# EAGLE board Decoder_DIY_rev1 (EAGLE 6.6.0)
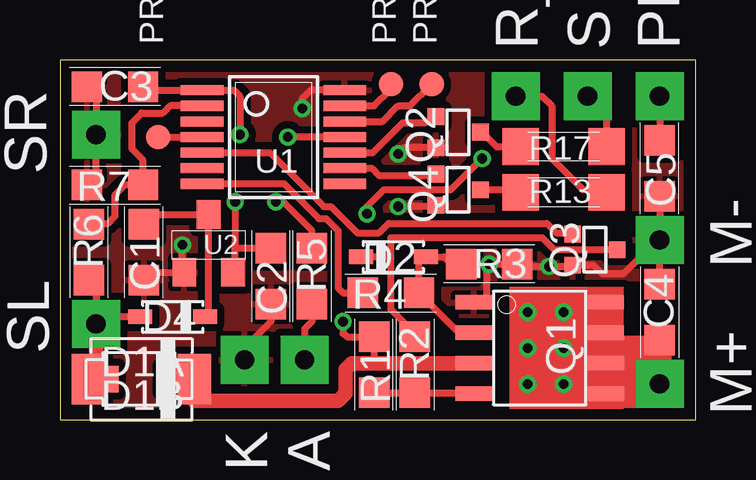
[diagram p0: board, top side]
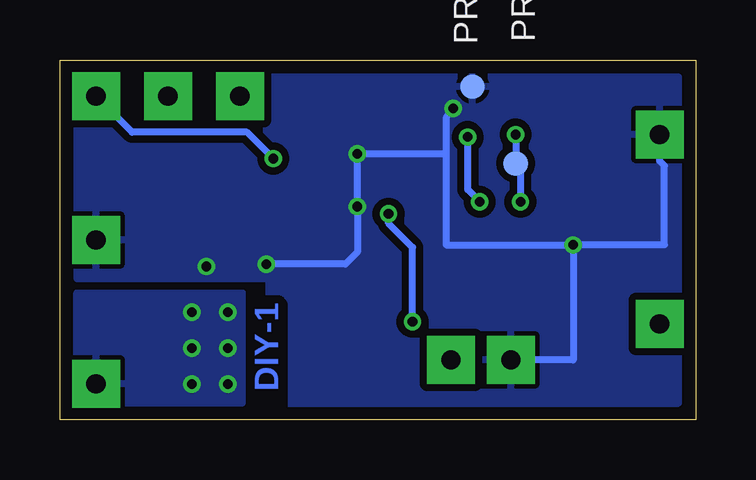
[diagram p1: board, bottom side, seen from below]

Size 26.5 x 15 mm. Coordinates in mm from the lower left corner, seen from the top.
Outline: 0,0 26.5,0 26.5,15 0,15 0,0
Copper layers (1*16): Top 0.035mm / dielectric 1.5mm / Bottom 0.035mm
Design rules "PCB-POOL Standard *": minimum track width 0.15mm, minimum drill 0.3mm, track to track 0.15mm, track to pad 0.15mm, pad to pad 0.15mm, via to via 0.15mm, smd to smd 0.15mm, copper to edge 0.3mm, drill to drill 0.2mm, minimum pad ring 0.2mm, minimum via ring 0.15mm, stop-mask expansion 0.075mm, vias tented up to drill 0.5mm, thermal gap 0.2mm
bRestrict: 2 lines

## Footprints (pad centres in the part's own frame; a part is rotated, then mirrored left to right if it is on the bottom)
LOETPAD_2X2_MM = drill 0.8 pad 2 square: P$1 0,0
0805 = smd 1.27 x 1.27: 1 -1.168,0; 2 1.168,0
SOD128 = smd 1.4 x 2.1: A -2.2,0; K 2.2,0
SOD123W = smd 1.1 x 1.1: A 1.4,0; K -1.4,0
SOD323 = smd 1 x 0.6: A 1.35,0; K -1.35,0
TESTPAD_RUND = smd 1.016 x 1.016: 1 0,0
SO8_COOLING = smd 0.61 x 1.524: 1 -1.905,-2.743; 2 -0.635,-2.743; 3 0.635,-2.743; 4 1.905,-2.743; 5 1.905,2.743; 6 0.635,2.743; 7 -0.635,2.743; 8 -1.905,2.743
SC70_FRANK = smd 0.7 x 0.7: 1 -0.65,-0.925; 2 0.65,-0.925; 3 0,0.925
1206 = smd 1.524 x 1.524: 1 1.792,0; 2 -1.79,0
TSSOP14 = smd 0.42 x 1.78: 1 -1.95,-2.97; 2 -1.3,-2.97; 3 -0.65,-2.97; 4 0,-2.97; 5 0.65,-2.97; 6 1.3,-2.97; 7 1.95,-2.97; 8 1.95,2.97; 9 1.3,2.97; 10 0.65,2.97; 11 0,2.97; 12 -0.65,2.97; 13 -1.3,2.97; 14 -1.95,2.97
SOT-23 = smd 0.991 x 1.194: 1 0,-1.27; 2 -1.016,1.143; 3 1.016,1.143

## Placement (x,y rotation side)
A  LOETPAD_2X2MM  [LOETPAD_2X2_MM]  10.2,2.5 0 top
C1  22u/16V/0805  [0805]  3.5,7 90 top
C2  100u/6,3V/0805  [0805]  8.8,6 90 top
C3  100n  [0805]  2.3,13.9 180 top
C4  100n  [0805]  25,4.5 270 top
C5  100n  [0805]  25,10.5 90 top
D1A  PMEG6030EP  [SOD128]  3.4,1.7 0 top
D1B  PMEG4020ER  [SOD123W]  3.3,1.7 180 top
D2  BAT760  [SOD323]  13.9,6.8 0 top
D4  BAT760  [SOD323]  4.7,4.3 180 top
K  LOETPAD_2X2MM  [LOETPAD_2X2_MM]  7.7,2.5 0 top
M+  LOETPAD_2X2MM  [LOETPAD_2X2_MM]  25,1.5 270 top
M-  LOETPAD_2X2MM  [LOETPAD_2X2_MM]  25,7.5 270 top
PLUS  LOETPAD_2X2MM  [LOETPAD_2X2_MM]  25,13.5 0 top
PROG_1  MCLR  [TESTPAD_RUND]  4.1,11.8 0 top
PROG_2  ICPDAT  [TESTPAD_RUND]  7.5,10.7 0 bottom
PROG_3  ICPDAT  [TESTPAD_RUND]  9.3,13.9 0 bottom
PROG_4  ICPDAT  [TESTPAD_RUND]  13.8,14 0 top
PROG_5  ICPCLK  [TESTPAD_RUND]  15.5,14 0 top
Q1  FDS8858CZ  [SO8_COOLING]  20,3 270 top
Q2  PDTC144EUA  [SC70_FRANK]  16.6,12 270 top
Q3  PDTC144EUA  [SC70_FRANK]  22.3,7.1 270 top
Q4  PDTC144EUA  [SC70_FRANK]  16.6,9.6 270 top
R1  1K  [0805]  13.1,2.3 90 top
R2  1K  [0805]  14.8,2.3 270 top
R3  18K  [0805]  17.9,6.5 180 top
R4  220R  [0805]  13.8,5.3 0 top
R5  390R  [0805]  10.5,6 270 top
R6  18K  [0805]  1.2,7 270 top
R7  10K  [0805]  2.3,9.8 0 top
R13  1K/1206  [1206]  21,9.5 180 top
R17  1K/1206  [1206]  21,11.4 180 top
R_B  LOETPAD_2X2MM  [LOETPAD_2X2_MM]  19,13.5 0 top
S  LOETPAD_2X2MM  [LOETPAD_2X2_MM]  22,13.5 0 top
SL  LOETPAD_2X2MM  [LOETPAD_2X2_MM]  1.5,4 0 top
SR  LOETPAD_2X2MM  [LOETPAD_2X2_MM]  1.5,11.9 0 top
U1  PIC16F1825-I/ST  [TSSOP14]  8.9,11.8 270 top
U2  MCP1703  [SOT-23]  6.2,7.3 180 top

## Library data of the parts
A D1A D1B K M+ M- PLUS Q1-Q4 R_B S SL SR U1 = Hobby
C1-C5 D2 D4 PROG_1-PROG_5 R1-R7 R13 R17 = SMD
U2 = SMD-IC

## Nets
!DATA!: R6.1 R7.2 U1.2
+5V: C2.2 C3.1 PROG_2.1 U1.1 U2.2
+15V: C5.2 D1A.K D1B.K PLUS.P$1 Q1.3 R1.2
BREMSE: R4.1 U1.7
D!: Q2.3 R17.1
GND: C1.1 C2.1 C3.2 C4.1 C5.1 K.P$1 M-.P$1 PROG_3.1 Q1.1 Q2.2 Q3.2 Q4.2 R3.1 R7.1 SR.P$1 U1.14 U2.3
IR_LED: R5.1 U1.11
LICHT: Q2.1 U1.10
M_PLUS: C4.2 M+.P$1 Q1.5 Q1.6 Q1.7 Q1.8
MOTOR: Q3.1 U1.5
N$1: C1.2 D4.K U2.1
N$2: PROG_5.1 U1.12
N$3: PROG_4.1 U1.13
N$4: R13.2 R_B.P$1
N$5: A.P$1 R5.2
N$6: D1A.A D1B.A D4.A R6.2 SL.P$1
N$9: R17.2 S.P$1
N$11: D2.A Q1.2 R3.2 R4.2
N$13: Q4.3 R13.1
N$16: D2.K Q3.3 R2.1
N$17: Q1.4 R1.1 R2.2
RüCK_BREMSLICHT: Q4.1 U1.9
VPP_!MCLR!: PROG_1.1 U1.4

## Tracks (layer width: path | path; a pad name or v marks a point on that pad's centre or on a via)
!DATA!
  Top 0.3: U1.2 4.6,13.1 4.3,12.8 3.4,12.8 3,12.4 3,11.3 3.47,10.83 R7.2 2.7,9.8 2.3,9.4 2.3,8.5 2,8.2 1.23,8.2 R6.1
+5V  (via drill 0.4)
  Top 0.3: U2.2 7.2,6.17 | C3.1 3.47,13.75 U1.1 7.25,13.75 7.5,13.5 v7.5,11.9 | U2.2 7.22,6.42 7.3,6.42 7.3,7.17 | 8.77,7.2 C2.2 7.3,7.17 | v7.3,9.1 7.3,7.4 7.3,7.17 | U2.2 7.3,6.07
  Bottom 0.3: v7.5,11.9 PROG_2.1 7.3,10.3 v7.3,9.1
+15V  (via drill 0.4)
  Top 0.3: D1B.K D1A.K | 13.1,2.37 R1.2 11.97,3.47 11.8,3.6 v11.8,4.1 | 16,2.4 16.8,2.3 16.84,2.3 16.9,2.37 | PLUS.P$1 C5.2 | v12.8,8.6 12.8,8.9 13.5,9.6 16.3,9.6 v17.6,10.9
  Top 0.6: D1A.K 5.6,0.8 11.6,0.8 11.9,1.1 11.9,2.1 12.16,2.37 13.1,2.37 16.9,2.37 Q1.3
  Bottom 0.3: v11.8,4.1 11.8,7.2 12.8,8.2 v12.8,8.6 | v17.6,10.9 18.7,12 23.5,12 PLUS.P$1
BREMSE
  Top 0.3: U1.7 9.35,9.85 10.8,8.4 11.1,8.4 11.6,7.9 11.6,5.5 11.8,5.3 R4.1
D!
  Top 0.3: Q2.3 17.6,12 18.2,11.4 R17.1
GND  (via drill 0.4)
  Top 0.3: 3.47,6.13 C1.1 3.52,6.16 U2.3 5.1,6.24 v5.1,7.3 | C2.1 8.8,4.1 7.7,3 K.P$1 | 1.3,13.93 C3.2 1.5,13.53 SR.P$1 1.5,10.17 R7.1 | U1.14 10.45,13.75 10.1,13.4 v10.1,13 | Q4.2 15.53,8.9 v14.1,8.9 | Q2.2 14.35,11.35 v14.1,11.1 | C4.1 M-.P$1 | C5.1 M-.P$1 | Q1.1 17.26,4.96 17.3,5 17.8,5 17.8,6.5 v17.9,6.5 R3.1 19.17,6.4 v20.4,6.4 21.32,6.4 Q3.2 22.25,6.45 22.6,6.1 23.5,6.1 24.9,7.5 M-.P$1
  Bottom 0.3: v5.1,7.3 5.1,2.5 K.P$1 | v5.1,7.3 1.3,7.3 1.3,10.6 1.5,10.8 SR.P$1 | v10.1,13 10.4,12.6 10.4,11.1 | 10.4,11.1 10.4,7.3 v5.1,7.3 | 10.4,11.1 v14.1,11.1 v14.1,8.9 14.1,7 14.6,6.5 v17.9,6.5
  pour Bottom (isolate 0.3): 0.7,14.3 25.8,14.3 25.8,5.9 17.8,5.9 17.8,0.7 0.7,0.7
  pour Top (isolate 0.3): 0.8,0.6 17.8,0.6 17.8,5.9 25.9,5.9 25.9,14.4 0.7,14.4 0.7,14.3 0.6,14.3 0.6,0.8
IR_LED  (via drill 0.4)
  Top 0.3: R5.1 10.5,7.9 9.3,9.1 v9,9.1 | U1.11 v9.5,11.8
  Bottom 0.3: v9,9.1 9.5,9.6 v9.5,11.8
LICHT
  Top 0.3: U1.10 13.05,11.15 14.3,12.4 15.22,12.4 Q2.1
M_PLUS  (via drill 0.4)
  Top 0.3: 24.5,1.2 24.5,1.5 M+.P$1 | 24.5,1 24.5,1.2 | 24.5,1.2 23.8,1.2 | Q1.5 22.74,1 22.8,1 | Q1.6 22.74,3 | 22.74,3 22.8,3 | 22.74,3 Q1.7 Q1.8
  Top 1: M+.P$1 25,3 | C4.2 25,3 | 25,3 22.8,3 | 23.8,3 23.8,1.2 | 22.8,1 24.5,1
  other vias: 19.5,4.5 21,4.5 19.5,3 21,3 19.5,1.5 21,1.5
  pour Bottom: 18.9,0.7 25.8,0.7 25.8,5.3 18.9,5.3
MOTOR
  Top 0.3: U1.5 8.75,11.15 11,8.9 11.3,8.9 12.4,7.8 13.3,7.8 13.7,8.2 20.3,8.2 20.7,7.8 21.32,7.8 Q3.1
N$1
  Top 0.3: C1.2 3.6,8.57 U2.1 6.2,4.4 6.1,4.3 D4.K
N$2
  Top 0.3: U1.12 13.45,12.45 14.1,13.1 14.6,13.1 PROG_5.1
N$3
  Top 0.3: U1.13 13.1,13.1 13.8,13.8 PROG_4.1
N$4
  Top 0.3: R13.2 21.8,9.6 20.5,10.9 20.5,13.1 20.1,13.5 R_B.P$1
N$5
  Top 0.3: R5.2 10.5,4.1 10.2,3.8 A.P$1
N$6
  Top 0.3: R6.2 1.5,5.83 SL.P$1 1.7,4.3 D4.A
  Top 0.6: 1.3,1.8 D1A.A | D1A.A D1B.A | SL.P$1 1.5,2 D1A.A
N$9
  Top 0.3: 22.7,11.51 R17.2 22.79,13.5 S.P$1
N$11
  Top 0.3: Q1.2 16.63,3.63 R4.2 14.97,6.62 D2.A 16,6.8 16.3,6.5 R3.2
N$13
  Top 0.3: Q4.3 18.9,9.6 R13.1
N$16
  Top 0.3: R2.1 14.8,3.6 13.8,4.6 13.8,6.8 | 13.8,6.8 D2.K | 13.8,6.8 13.8,7.6 20.1,7.6 20.6,7.1 Q3.3
N$17
  Top 0.3: R1.1 R2.2 17.12,1.13 Q1.4
RüCK_BREMSLICHT
  Top 0.3: U1.9 13,10.5 13.3,10.2 15.53,10.2 Q4.1
VPP_!MCLR!
  Top 0.3: PROG_1.1 U1.4

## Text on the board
Bottom: DIY-1
Document: Decoder DIY Rev.1 / / SL Slot Links / SR Slot Rechts / A IR-LED Anode / K IR-LED Kathode / R_B LED (2 in Reihe) Rücklicht Kathode / S LED (2 in Reihe) Scheinwerfer Kathode / PLUS LED Rücklicht und Scheinwerfer Anode / / PROG_1 PICkit3 Pin1 !MCLR! / PROG_2 PICkit3 Pin2 5V / PROG_3 PICkit3 Pin3 GND / PROG_4 PICkit3 Pin4 DAT / PROG_5 PICkit3 Pin5 CLK / n.c. PICkit3 Pin6 frei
